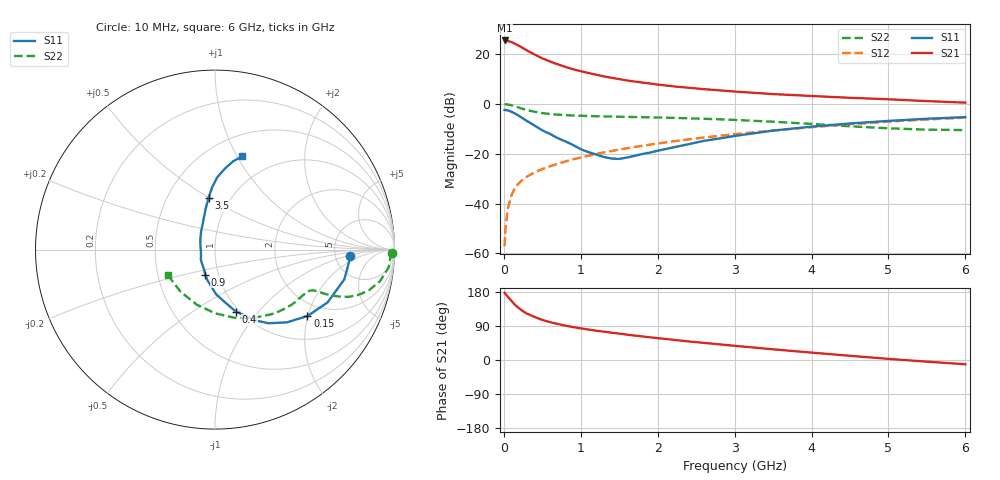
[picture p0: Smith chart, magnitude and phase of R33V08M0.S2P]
! SIEMENS Small Signal Semiconductors
! BFR181
! Si NPN RF Bipolar Junction Transistor in SOT23
! VCE = 3 V  IC = 8 mA
! Common Emitter S-Parameters:  May  1996
# GHz  S  MA  R  50
!  f  S11  S21  S12  S22
! GHz  MAG  ANG  MAG  ANG  MAG  ANG  MAG  ANG
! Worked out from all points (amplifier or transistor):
!   36 points, 10 MHz to 6 GHz, reference 50 ohm
!   highest |S21| = 25.4 dB at 10 MHz (marker M1)
!   |S21| within 3 dB of that: start of sweep to 245.9 MHz
!   unconditionally stable (mu >= 1): 877.6 MHz to 2.718 GHz
!   at 250 MHz: K = 0.55, MSG = 26.3 dB, |S12| = -30.2 dB
!   at 1.4 GHz: K = 1.06, MAG = 13.2 dB, |S12| = -18.9 dB
!   at 6 GHz: K = 0.86, MSG = 3.0 dB, |S12| = -5.5 dB
!   S11 on the Smith chart (normalised r, x): 10 MHz: 6.98, -1.07; 150 MHz: 1.61, -1.99; 400 MHz: 0.96, -0.77; 900 MHz: 0.86, -0.25; 3.5 GHz: 0.79, +0.50; 6 GHz: 0.72, +1.05
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0.01  0.7545 -2.5  18.67 177.2  0.0014 94.3  0.9872 -1.0
0.02  0.7495 -5.5  18.35 174.5  0.0031 86.9  0.9788 -2.3
0.05  0.7395 -12.9  18.25 167.3  0.0077 82.9  0.9729 -5.8
0.1  0.6927 -25.2  17.34 155.8  0.0148 78.5  0.9355 -10.9
0.15  0.6343 -35.7  15.87 144.7  0.0214 73.1  0.8859 -14.9
0.2  0.5701 -45.3  14.49 136.1  0.026 71.2  0.8362 -17.6
0.25  0.5073 -54.0  13.11 128.5  0.0308 68.2  0.7887 -19.5
0.3  0.4547 -60.2  11.78 122.5  0.0347 68.5  0.7496 -20.5
0.4  0.3662 -71.2  9.757 113.6  0.0423 66.8  0.6942 -21.6
0.5  0.2942 -80.0  8.175 105.6  0.0493 66.8  0.653 -22.0
0.6  0.2488 -88.6  7.078 99.9  0.0559 67.1  0.6252 -22.1
0.7  0.2057 -95.9  6.211 95.1  0.0628 67.5  0.6073 -22.3
0.9  0.1496 -111.2  4.945 86.8  0.0773 67.9  0.5843 -22.9
1.1  0.1075 -131.7  4.156 80.4  0.0911 68.5  0.5694 -24.2
1.3  0.0858 -155.1  3.556 74.7  0.1061 68.3  0.5589 -25.7
1.6  0.0838 165.8  2.948 66.9  0.1288 67.5  0.5476 -28.7
2.2  0.1336 124.6  2.245 53.4  0.1767 64.8  0.5231 -36.4
2.8  0.2018 106.8  1.867 41.4  0.2282 60.7  0.4902 -45.8
3.5  0.2906 97.1  1.57 28.2  0.2922 54.7  0.4379 -60.2
4.5  0.4045 88.1  1.323 11.1  0.3905 43.9  0.3547 -89.9
5.5  0.5025 78.4  1.135 -4.4  0.4863 31.0  0.3031 -129.5
6  0.5416 73.6  1.057 -11.3  0.5292 23.9  0.2984 -151.5
